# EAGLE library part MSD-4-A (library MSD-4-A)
Memory Card Connectors 9 Positions, Push In, Auto Eject Out, SMT, 1.8 mm Height Above Board, Source: Datasheet
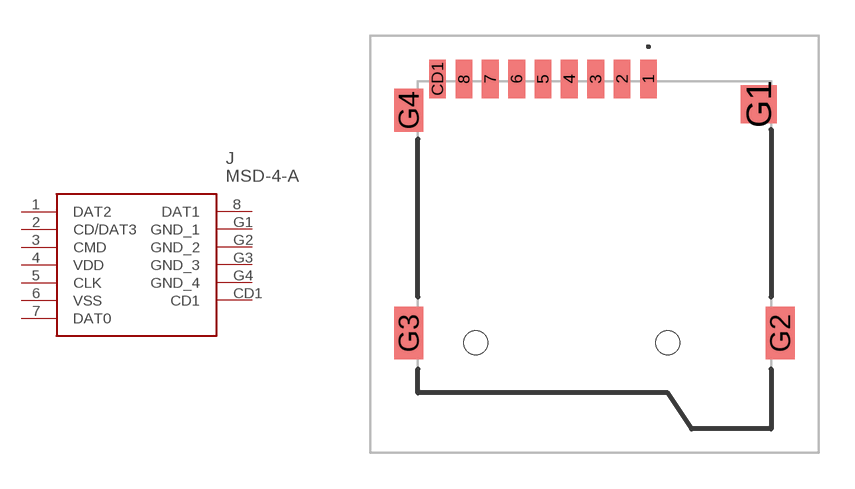
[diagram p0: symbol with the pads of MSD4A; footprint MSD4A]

Designator prefix J

## MSD-4-A (Description: Memory Card Connectors 9 Positions, Push In, Auto Eject Out, SMT, 1.8 mm Height Above Board,; Height: 2mm; Manufacturer_Name: Same Sky; Manufacturer_Part_Number: MSD-4-A; Mouser_Part_Number: 179-MSD-4-A; Mouser_Price-Stock: https://www.mouser.co.uk/ProductDetail/Same-Sky/MSD-4-A?qs=Z%252BL2brAPG1Jll%252BQTi%252Btupg%3D%3D)  [MSD4A]
1  DAT2
2  CD/DAT3
3  CMD
4  VDD
5  CLK
6  VSS
7  DAT0
8  DAT1
CD1  CD1
G1  GND_1
G2  GND_2
G3  GND_3
G4  GND_4

## Footprint MSD4A (pad centres in mm)
MSD-4-A-2
smd 0.7 x 1.6: 1 2.25,6.9; 2 1.15,6.9; 3 0.05,6.9; 4 -1.05,6.9; 5 -2.15,6.9; 6 -3.25,6.9; 7 -4.35,6.9; 8 -5.45,6.9; CD1 -6.55,6.9
smd 1.5 x 1.6: G1 6.85,5.85
smd 1.2 x 2.2: G2 7.75,-3.7; G3 -7.75,-3.7
smd 1.2 x 1.8: G4 -7.75,5.6
hole 1 at 3.05,-4.1
hole 1 at -4.95,-4.1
